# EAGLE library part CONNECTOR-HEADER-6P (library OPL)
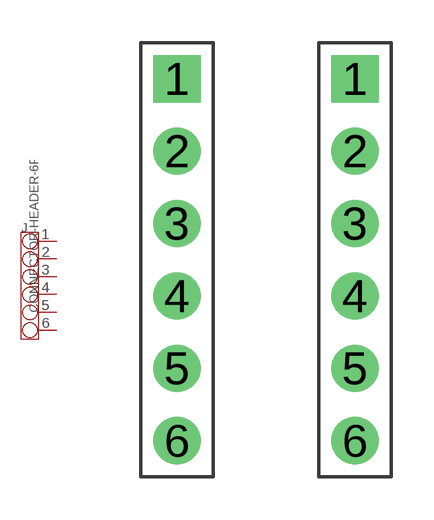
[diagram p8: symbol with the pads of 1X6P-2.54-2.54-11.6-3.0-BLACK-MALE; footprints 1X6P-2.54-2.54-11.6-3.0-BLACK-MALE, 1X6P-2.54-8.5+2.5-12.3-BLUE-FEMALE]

Designator prefix J

## CONNECTOR-HEADER-6P-3460650P1  [1X6P-2.54-2.54-11.6-3.0-BLACK-MALE]
1  1
2  2
3  3
4  4
5  5
6  6

## CONNECTOR-HEADER-6P-3461250P1  [1X6P-2.54-8.5+2.5-12.3-BLUE-FEMALE]
Pads as for 1X6P-2.54-2.54-11.6-3.0-BLACK-MALE

## CONNECTOR-HEADER-6P-3460270P1  [1X6P-2.54-8.5-BLACK-FEMALE]
Pads as for 1X6P-2.54-2.54-11.6-3.0-BLACK-MALE

## CONNECTOR-HEADER-6P-3460540P1  [1X6P-2.54-8.5-WHITE-FEMALE]
Pads as for 1X6P-2.54-2.54-11.6-3.0-BLACK-MALE

## Footprint 1X6P-2.54-2.54-11.6-3.0-BLACK-MALE (pad centres in mm)
drill 0.889 pad 1.651 square: 1 0,6.35
drill 0.889 pad 1.651: 2 0,3.81; 3 0,1.27; 4 0,-1.27; 5 0,-3.81; 6 0,-6.35

## Footprint 1X6P-2.54-8.5+2.5-12.3-BLUE-FEMALE (pad centres in mm)
drill 0.889 pad 1.651 square: 1 0,6.35
drill 0.889 pad 1.651: 2 0,3.81; 3 0,1.27; 4 0,-1.27; 5 0,-3.81; 6 0,-6.35

## Footprint 1X6P-2.54-8.5-BLACK-FEMALE (pad centres in mm)
drill 0.889 pad 1.651 square: 1 0,6.35
drill 0.889 pad 1.651: 2 0,3.81; 3 0,1.27; 4 0,-1.27; 5 0,-3.81; 6 0,-6.35

## Footprint 1X6P-2.54-8.5-WHITE-FEMALE (pad centres in mm)
drill 0.889 pad 1.651 square: 1 0,6.35
drill 0.889 pad 1.651: 2 0,3.81; 3 0,1.27; 4 0,-1.27; 5 0,-3.81; 6 0,-6.35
